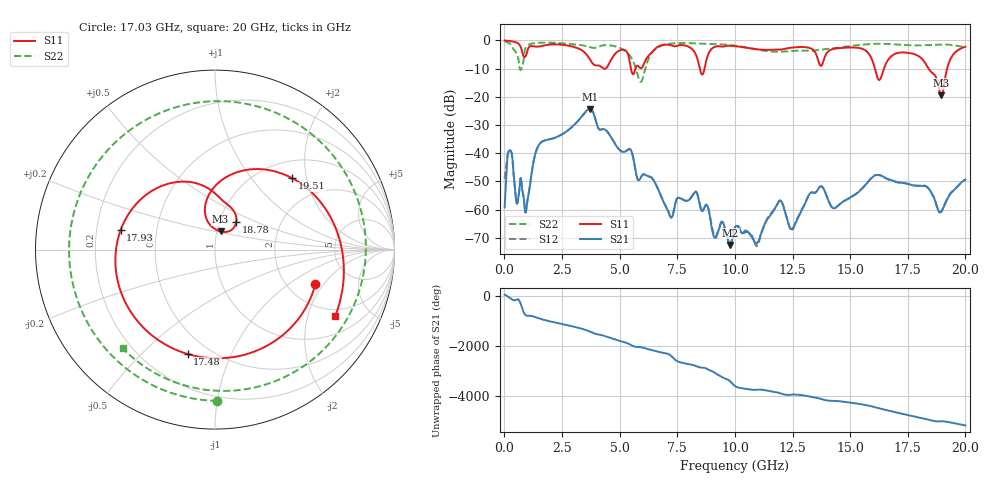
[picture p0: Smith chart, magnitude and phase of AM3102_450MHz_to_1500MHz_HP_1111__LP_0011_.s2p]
!Agilent Technologies,E8364B,MY43040894,A.07.50.67
!Agilent E8364B: A.07.50.67
!Date: Thursday, January 11, 2018 06:49:20
!Correction: S11(Full 2 Port(1,2))
!S21(Full 2 Port(1,2))
!S12(Full 2 Port(1,2))
!S22(Full 2 Port(1,2))
!S2P File: Measurements: S11, S21, S12, S22:
# Hz S  dB  R 50
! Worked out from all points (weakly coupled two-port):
!   1601 points, 10 MHz to 20 GHz, reference 50 ohm
!   highest |S21| = -24.30 dB at 3.708 GHz (marker M1); lowest = -72.5 dB at 9.805 GHz (marker M2)
!   lowest |S11| = -19.5 dB at 18.95 GHz (marker M3), VSWR 1.24, Z = 52.1 + j10.7 ohm
!   |S11| at or under -10 dB: 8.477 GHz to 8.684 GHz (207.1 MHz wide, 2.41 % of centre); 16.07 GHz to 16.47 GHz (396.1 MHz wide, 2.43 % of centre); 18.4 GHz to 19.21 GHz (809.8 MHz wide, 4.31 % of centre)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
!   |S22| runs from -14.7 to -0.4 dB; largest |S21 - S12| = 0.0026
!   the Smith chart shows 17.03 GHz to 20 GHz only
!   S11 on the Smith chart (normalised r, x): 17.03 GHz: 2.83, -1.65; 17.48 GHz: 0.38, -0.70; 17.93 GHz: 0.30, +0.09; 18.78 GHz: 1.20, +0.38; 19.51 GHz: 1.36, +1.65; 20 GHz: 1.68, -3.01
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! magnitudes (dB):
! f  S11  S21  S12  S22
! 10 MHz  -0.1  -59.2  -49.1  -0.4
! 234.9 MHz  -0.3  -38.9  -38.9  -1.2
! 947 MHz  -5.2  -60.3  -60.0  -2.3
! 1.497 GHz  -2.2  -37.1  -37.1  -0.9
! 3.346 GHz  -3.5  -27.1  -27.1  -1.7
! 3.708 GHz  -6.7  -24.3  -24.3  -2.4
! 5.907 GHz  -9.9  -48.8  -48.8  -14.7
! 6.682 GHz  -2.2  -53.0  -53.0  -2.4
! 9.805 GHz  -1.9  -72.5  -72.3  -1.7
! 10.01 GHz  -2.1  -66.3  -66.2  -1.9
! 10.97 GHz  -3.2  -71.9  -72.8  -3.3
! 11.95 GHz  -3.3  -56.7  -56.8  -4.0
! 12.48 GHz  -2.6  -67.1  -67.2  -3.8
! 13.34 GHz  -3.1  -53.9  -53.8  -3.8
! 16.68 GHz  -6.6  -49.3  -49.3  -1.3
! 17.03 GHz  -4.6  -50.3  -50.3  -1.5
! 17.48 GHz  -4.4  -50.8  -50.8  -1.7
! 17.93 GHz  -5.4  -51.5  -51.6  -1.8
! 18.78 GHz  -14.3  -59.1  -59.2  -1.5
! 18.95 GHz  -19.5  -60.8  -60.6  -1.5
! 19.51 GHz  -4.6  -53.0  -52.9  -1.8
! 20 GHz  -2.3  -49.4  -49.4  -2.5
